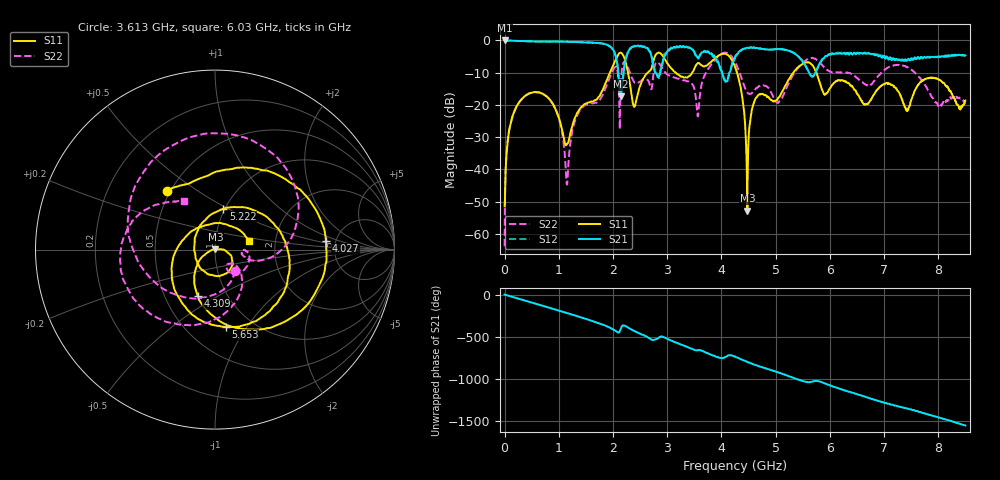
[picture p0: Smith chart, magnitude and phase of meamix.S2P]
!Agilent Technologies,E5071B,MY42402595,A.08.01
!Date: Mon Jan 01 23:43:58 2001
!Data & Calibration Information:
!Freq	S11:SOLT2(ON)	S21:SOLT2(ON)	S12:SOLT2(ON)	S22:SOLT2(ON)
# Hz S dB R 50
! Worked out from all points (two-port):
!   1601 points, 300 kHz to 8.5 GHz, reference 50 ohm
!   highest |S21| = 0.01 dB at 300 kHz (marker M1); lowest = -17.3 dB at 2.141 GHz (marker M2)
!   |S21| within 3 dB of the highest: start of sweep to 2.007 GHz; 4.365 GHz to 5.207 GHz (841.5 MHz wide, 17.6 % of centre)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
!   lowest |S11| = -52.8 dB at 4.479 GHz (marker M3), VSWR 1.00, Z = 50.2 + j0.0623 ohm
!   |S11| at or under -10 dB: start of sweep to 1.942 GHz; 4.288 GHz to 5.325 GHz (1.037 GHz wide, 21.6 % of centre); 5.753 GHz to end of sweep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
!   |S22| runs from -63.8 to -3.8 dB; largest |S21 - S12| = 0.065
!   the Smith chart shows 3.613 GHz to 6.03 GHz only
!   S11 on the Smith chart (normalised r, x): 3.613 GHz: 0.48, +0.38; 4.027 GHz: 4.15, +0.66; 4.309 GHz: 0.73, -0.41; 5.222 GHz: 0.98, +0.47; 5.653 GHz: 0.76, -0.81; 6.03 GHz: 1.46, +0.15
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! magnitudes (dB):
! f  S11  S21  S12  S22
! 300 kHz  -51.4  0.0  0.0  -63.8
! 79.98 MHz  -28.3  -0.1  0.0  -28.2
! 287.2 MHz  -18.8  -0.2  -0.2  -18.7
! 860.9 MHz  -19.0  -0.3  -0.4  -19.0
! 1.148 GHz  -32.2  -0.4  -0.4  -44.7
! 1.419 GHz  -20.6  -0.6  -0.6  -21.0
! 1.971 GHz  -8.8  -2.2  -2.2  -10.2
! 2.141 GHz  -3.8  -17.3  -17.2  -15.2
! 2.396 GHz  -20.6  -1.7  -1.8  -13.0
! 2.837 GHz  -3.8  -11.5  -10.9  -6.9
! 3.613 GHz  -7.5  -4.4  -4.2  -15.7
! 4.027 GHz  -4.2  -11.0  -10.9  -3.9
! 4.25 GHz  -8.1  -5.2  -5.3  -6.7
! 4.309 GHz  -11.2  -3.8  -3.9  -8.9
! 4.479 GHz  -52.8  -2.2  -2.3  -16.2
! 4.649 GHz  -17.6  -2.4  -2.3  -14.7
! 5.222 GHz  -12.7  -3.1  -3.1  -13.9
! 5.653 GHz  -7.2  -10.9  -10.9  -5.5
! 5.669 GHz  -7.5  -11.2  -11.1  -5.4
! 6.03 GHz  -14.1  -4.2  -4.1  -9.8
! 7.087 GHz  -13.4  -5.9  -5.3  -8.3
! 8.5 GHz  -18.6  -4.7  -4.7  -19.7
